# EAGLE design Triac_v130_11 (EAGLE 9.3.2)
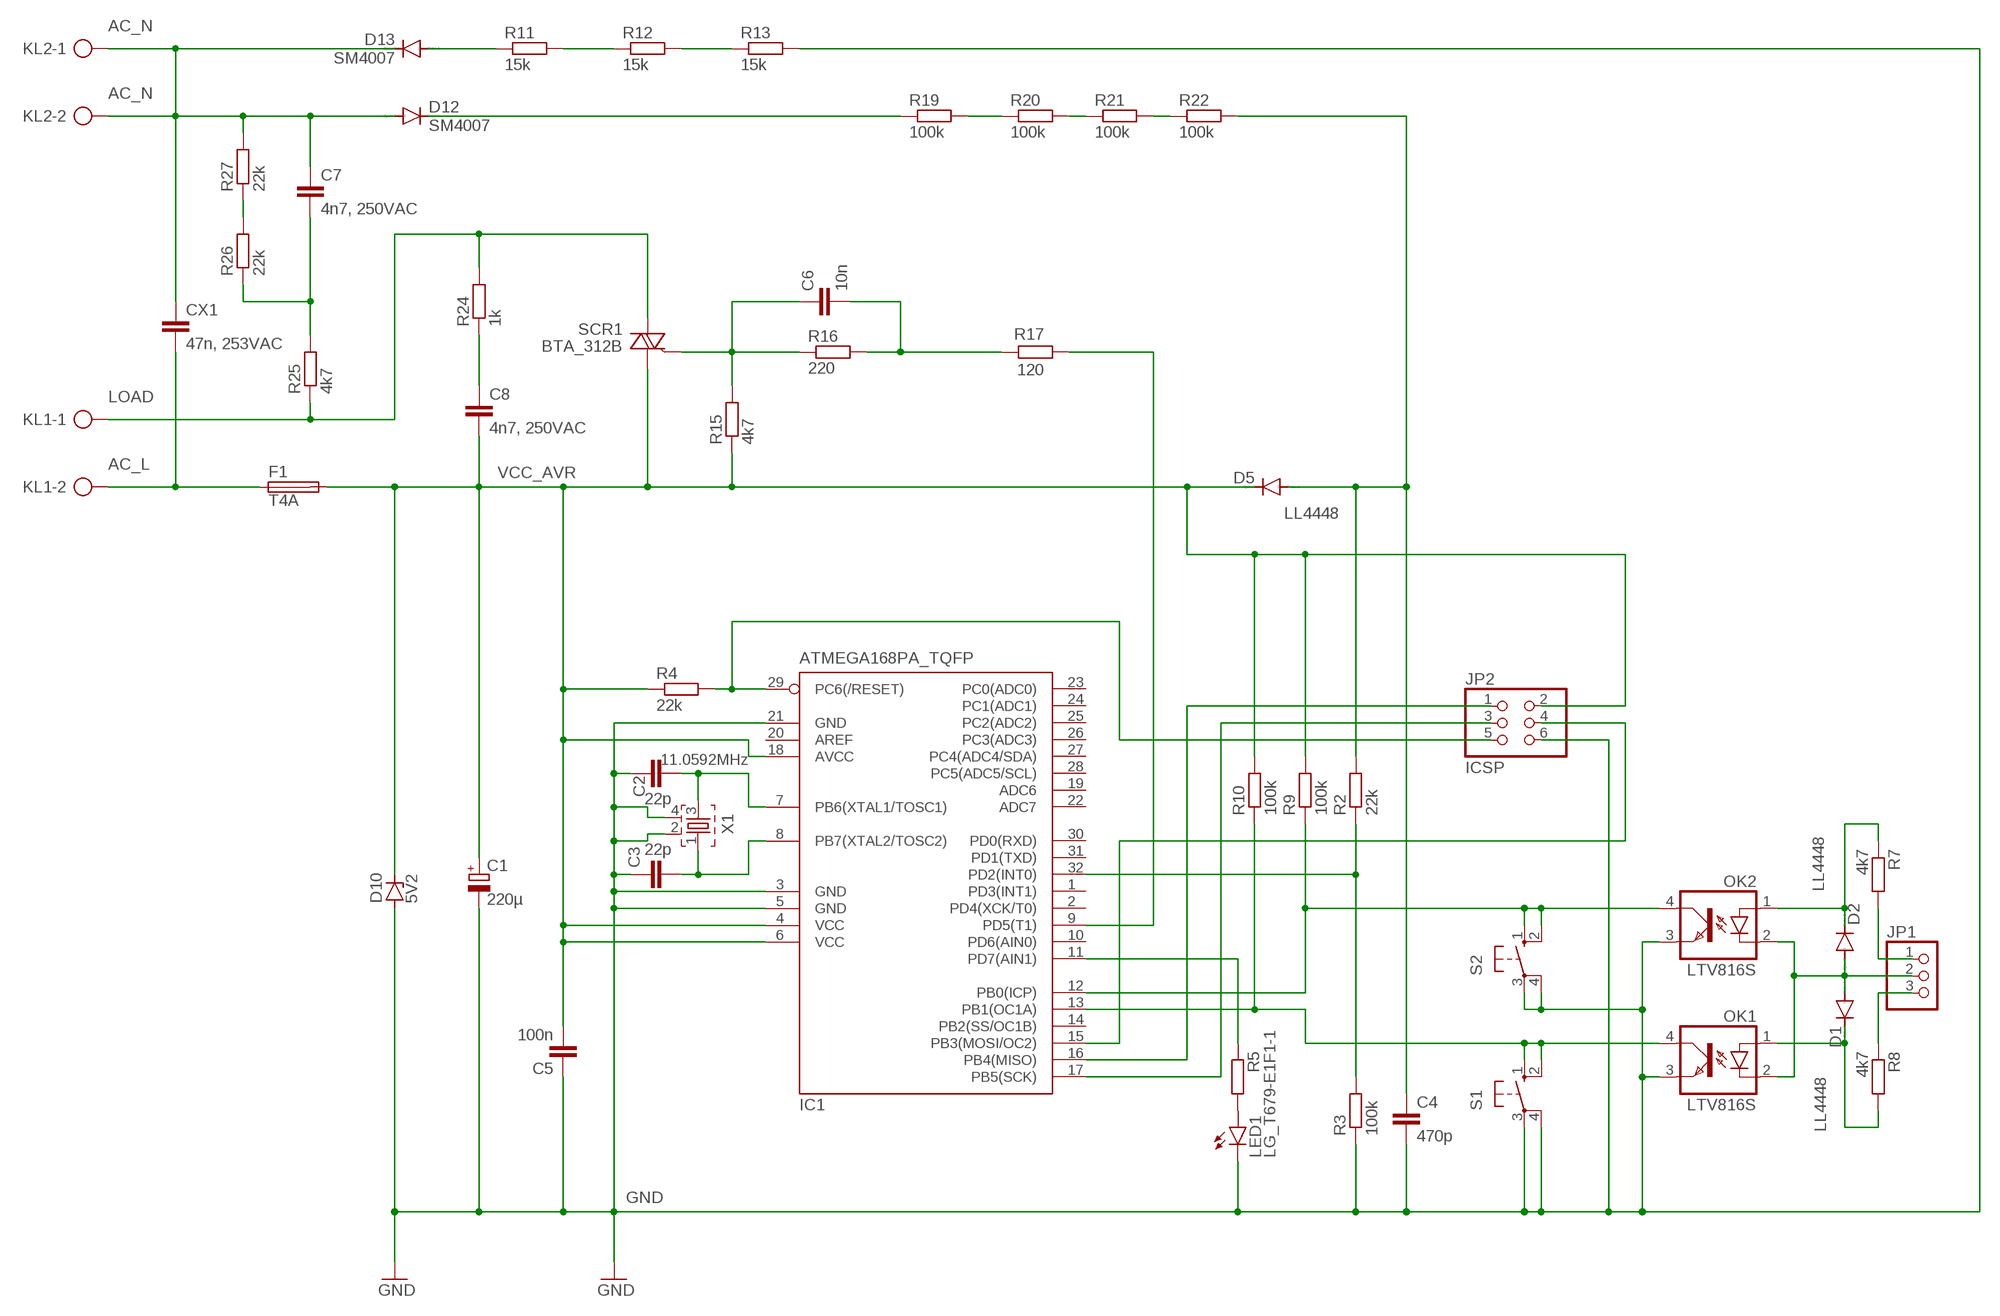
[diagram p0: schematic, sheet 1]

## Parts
C1  220µ  CPOL-EU153CLV-0605  [153CLV-0605]
C2  22p  C-EUC0805  [C0805]
C3  22p  C-EUC0805  [C0805]
C4  470p  C-EUC0805  [C0805]
C5  100n  C-EUC0805  [C0805]
C6  10n  C-EUC0805K  [C0805K]
C7  4n7, 250VAC  C5/3  [C5B3]
C8  4n7, 250VAC  C5/3  [C5B3]
CX1  47n, 253VAC  XC_03  [XC22B6]
D1  LL4448  [SOD80C]
D2  LL4448  [SOD80C]
D5  LL4448  [SOD80C]
D10  5V2  ZENER-DIODESOD80C  [SOD80C]
D12  SM4007  DIODE-DO214AA  [DO214AA]
D13  SM4007  DIODE-DO214AA  [DO214AA]
F1  T4A  SHK20QPADS  [SHK20Q]
IC1  ATMEGA168PA_TQFP  MEGA8-AI  [TQFP32-08]
JP1  PINHD-1X3  [1X03]
JP2  ICSP  PIN2X3  [2X03]
KL1  2pole-7.5mm  KL2_75  [KL2-75]
KL2  KL2_75  [KL2-75]
LED1  LG_T679-E1F1-1  [PLCC2]
OK1  LTV816S  [DIL4-SMD]
OK2  LTV816S  [DIL4-SMD]
R2  22k  R-EU_R0805  [R0805]
R3  100k  R-EU_R0805  [R0805]
R4  22k  R-EU_R0805  [R0805]
R5  R-EU_R0805  [R0805]
R7  4k7  R-EU_R0805  [R0805]
R8  4k7  R-EU_R0805  [R0805]
R9  100k  R-EU_R0805  [R0805]
R10  100k  R-EU_R0805  [R0805]
R11  15k  R-EU_MELF0207R  [MINI_MELF-0207R]
R12  15k  R-EU_MELF0207R  [MINI_MELF-0207R]
R13  15k  R-EU_MELF0207R  [MINI_MELF-0207R]
R15  4k7  R-EU_R0805  [R0805]
R16  220  R-EU_R0805  [R0805]
R17  120  R-EU_R0805  [R0805]
R19  100k  R-EU_R0805  [R0805]
R20  100k  R-EU_R0805  [R0805]
R21  100k  R-EU_R0805  [R0805]
R22  100k  R-EU_R0805  [R0805]
R24  1k  R-EU_MELF0207R  [MINI_MELF-0207R]
R25  4k7  R-EU_MELF0207R  [MINI_MELF-0207R]
R26  22k  R-EU_MELF0207R  [MINI_MELF-0207R]
R27  22k  R-EU_MELF0207R  [MINI_MELF-0207R]
S1  10-XX  [B3F-10XX]
S2  10-XX  [B3F-10XX]
SCR1  BTA_312B  [D2PACK]
X1  11.0592MHz  406_NEW  [CTS406]

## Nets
AC_L: CX1.2 F1.1A F1.1B KL1.2
AC_N: C7.1 CX1.1 D12.A D13.C KL2.1 KL2.2 R27.2
GND: C1.- C2.1 C3.1 C4.2 C5.1 D10.A IC1.3(GND) IC1.5(GND) IC1.21(GND) JP2.6 LED1.C OK1.3(EMIT) OK2.3(EMIT) R3.1 R13.2 S1.3(P) S1.4(P1) S2.3(P) S2.4(P1) X1.2 X1.4
LOAD: KL1.1 R24.2 R25.1 SCR1.T2(A2)
N$1: C2.2 IC1.7(PB6(XTAL1/TOSC1)) X1.3
N$3: IC1.11(PD7(AIN1)) R5.1
N$4: R26.2 R27.1
N$5: D13.A R11.1
N$6: R11.2 R12.1
N$7: R12.2 R13.1
N$8: C6.1 R15.2 R16.1 SCR1.G
N$9: D12.C R19.1
N$10: R19.2 R20.1
N$11: R20.2 R21.1
N$12: R21.2 R22.1
N$13: C6.2 R16.2 R17.2
N$14: C3.2 IC1.8(PB7(XTAL2/TOSC2)) X1.1
N$15: C7.2 R25.2 R26.1
N$16: C4.1 D5.A R2.2 R22.2
N$17: IC1.29(PC6(/RESET)) JP2.5 R4.2
N$18: C8.1 R24.1
N$19: IC1.12(PB0(ICP)) OK2.4(COL) R9.1 S2.1(S) S2.2(S1)
N$23: IC1.17(PB5(SCK)) JP2.3
N$24: LED1.A R5.2
N$25: IC1.9(PD5(T1)) R17.1
N$26: IC1.13(PB1(OC1A)) OK1.4(COL) R10.1 S1.1(S) S1.2(S1)
N$27: JP1.1 R7.2
N$28: IC1.32(PD2(INT0)) R2.1 R3.2
N$29: D2.C OK2.1(A) R7.1
N$30: JP1.3 R8.1
N$31: D1.C OK1.1(A) R8.2
N$32: IC1.16(PB4(MISO)) JP2.1
N$34: D1.A D2.A JP1.2 OK1.2(C) OK2.2(C)
N$36: IC1.15(PB3(MOSI/OC2)) JP2.4
VCC_AVR: C1.+ C5.2 C8.2 D5.C D10.C F1.2A F1.2B IC1.4(VCC) IC1.6(VCC) IC1.18(AVCC) JP2.2 R4.1 R9.2 R10.2 R15.1 SCR1.T1(A1)
Unconnected: IC1.1(PD3(INT1)) IC1.2(PD4(XCK/T0)) IC1.10(PD6(AIN0)) IC1.14(PB2(SS/OC1B)) IC1.19(ADC6) IC1.20(AREF) IC1.22(ADC7) IC1.23(PC0(ADC0)) IC1.24(PC1(ADC1)) IC1.25(PC2(ADC2)) IC1.26(PC3(ADC3)) IC1.27(PC4(ADC4/SDA)) IC1.28(PC5(ADC5/SCL)) IC1.30(PD0(RXD)) IC1.31(PD1(TXD))

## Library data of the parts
C1 = rcl:CPOL-EU: POLARIZED CAPACITOR, European symbol; SPICEPREFIX: C
C2-C6 = rcl:C-EU: CAPACITOR, European symbol; SPICEPREFIX: C
C7 C8 = capacitor-wima:C: CAPACITOR
CX1 = MY_CX:XC_03: Device XC_03
D1 D2 D5 = My_Diode:LL4448
D10 = diode:ZENER-DIODE: Z-Diode
D12 D13 = diode:DIODE-: DIODE
F1 = MY_Fuse:SHK20Q: FUSE HOLDER
IC1 = atmel:MEGA8: MICROCONTROLLER 8 Kbytes FLASH, 1 kbytes SRAM, 512 bytes EEPROM, USART, 6-channel 10 bit ADC, 2-channel 8 bit ADC Pin compatible with Atmega48, ATMega88, ATMega168 Source: avr.lbr; MPN: ATMEGA8-16AU; OC_FARNELL: 9171371; OC_NEWARK: 73M8863
JP1 = pinhead:PINHD-1X3: PIN HEADER
JP2 = pinhead_2x3:PIN2X3
KL1 KL2 = MY_Clamp_1:KL2_75: 2-pole Screw Terminal
LED1 = led:*_T679-?-1: LC TOPLED® Low Current LED; COLOR: green
OK1 OK2 = optocoupler:LTV816: OPTO COUPLER Source: LITEON, LTV816.pdf
R2-R5 R7-R13 R15-R17 R19-R22 R24-R27 = rcl:R-EU_: RESISTOR, European symbol; SPICEPREFIX: R
S1 S2 = switch-omron:10-XX: OMRON SWITCH; MPN: B3F-1000; OC_FARNELL: 176432; OC_NEWARK: 36M3542
SCR1 = BTA312B:BTA_312B
X1 = My_Crystal1:406_NEW

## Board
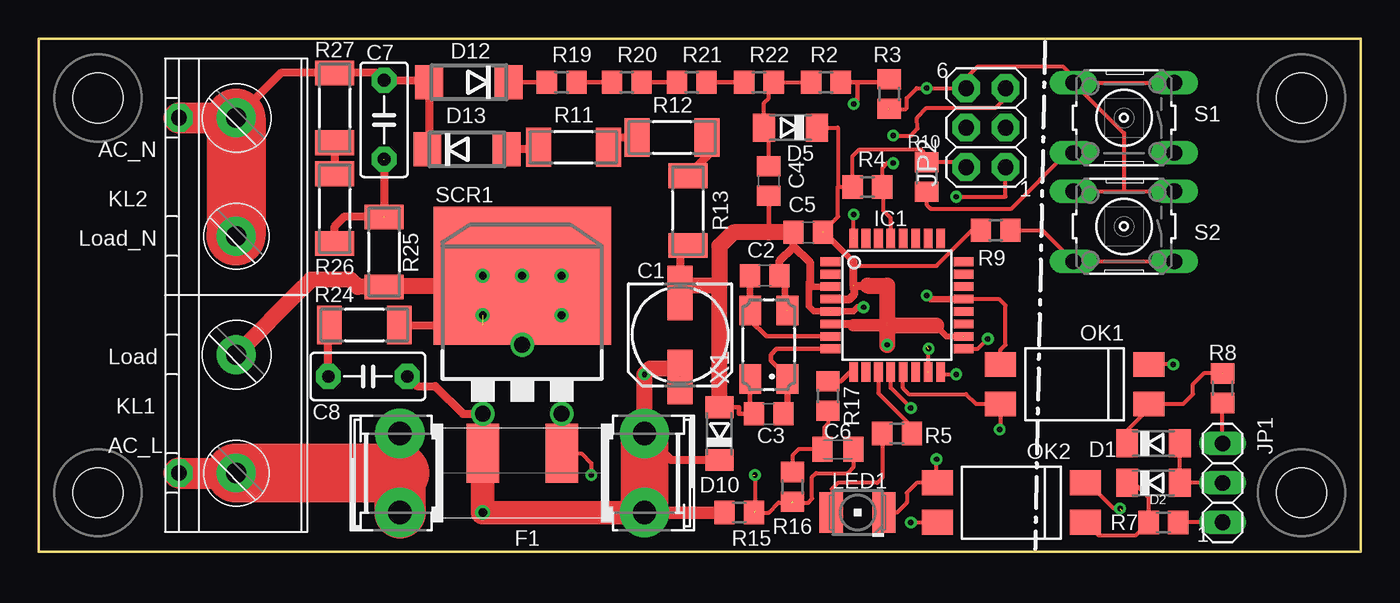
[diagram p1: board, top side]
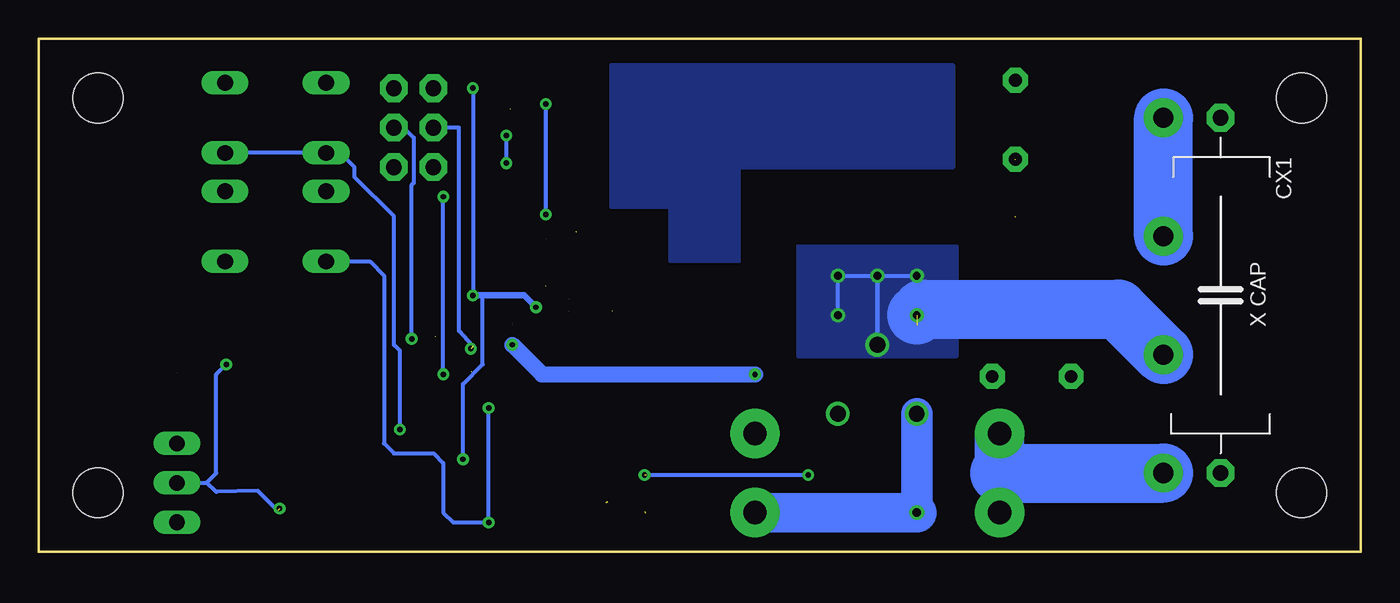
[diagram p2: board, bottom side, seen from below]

Size 85.09 x 33.02 mm. Coordinates in mm from the lower left corner, seen from the top.
Outline: 0,33.02 0,0 85.09,0 85.09,33.02 0,33.02
Copper layers (1*16): Top 0.035mm / dielectric 1.5mm / Bottom 0.035mm
Design rules "default *": minimum track width 10mil, minimum drill 0.35mm, track to track 6mil, track to pad 6mil, pad to pad 6mil, via to via 6mil, smd to smd 6mil, copper to edge 30mil, drill to drill 6mil, minimum pad ring 10mil, minimum via ring 8mil, stop-mask expansion 6mil, vias tented up to drill 0mil, thermal gap 10mil
Holes 3.2 mm at 81.28,3.81 81.28,29.21 3.81,3.81 3.81,29.21

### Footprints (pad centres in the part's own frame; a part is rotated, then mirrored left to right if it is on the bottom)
153CLV-0605 = smd 3.5 x 1.6: + 2.7,0; - -2.7,0
C0805 = smd 1.3 x 1.5: 1 -0.95,0; 2 0.95,0
C0805K = smd 1.3 x 1.6: 1 -1,0; 2 1,0
C5B3 = drill 0.813 pad 1.6 octagon: 1 -2.54,0; 2 2.54,0
XC22B6 = drill 1.016 pad 1.778 octagon: 1 -11.43,0; 2 11.43,0
SOD80C = smd 1.4 x 1.8: A 1.7,0; C -1.7,0
DO214AA = smd 1.8 x 2.2: A 2.55,0; C -2.55,0
SHK20Q = drill 1.5 pad 3.175: 1A -7.874,2.54; 1B -7.874,-2.54; 2A 7.874,2.54; 2B 7.874,-2.54
TQFP32-08 = smd 1.27 x 0.559: 1 -4.293,2.8; 2 -4.293,2; 3 -4.293,1.2; 4 -4.293,0.4; 5 -4.293,-0.4; 6 -4.293,-1.2; 7 -4.293,-2; 8 -4.293,-2.8; 17 4.293,-2.8; 18 4.293,-2; 19 4.293,-1.2; 20 4.293,-0.4; 21 4.293,0.4; 22 4.293,1.2; 23 4.293,2; 24 4.293,2.8 | smd 0.559 x 1.27: 9 -2.8,-4.293; 10 -2,-4.293; 11 -1.2,-4.293; 12 -0.4,-4.293; 13 0.4,-4.293; 14 1.2,-4.293; 15 2,-4.293; 16 2.8,-4.293; 25 2.8,4.293; 26 2,4.293; 27 1.2,4.293; 28 0.4,4.293; 29 -0.4,4.293; 30 -1.2,4.293; 31 -2,4.293; 32 -2.8,4.293
1X03 = drill 1.016 long: 1 -2.54,0; 2 0,0; 3 2.54,0
2X03 = drill 1.016 pad 1.778 octagon: 1 -2.54,-1.27; 2 -2.54,1.27; 3 0,-1.27; 4 0,1.27; 5 2.54,-1.27; 6 2.54,1.27
KL2-75 = drill 1.3 pad 2.5: 1 -3.81,0; 2 3.81,0
PLCC2 = smd 2.6 x 1.5: A 0,1.7; C 0,-1.7
DIL4-SMD = smd 1.6 x 2: 1 -1.27,-4.77; 2 1.27,-4.77; 3 1.27,4.77; 4 -1.27,4.77
R0805 = smd 1.3 x 1.5: 1 -0.95,0; 2 0.95,0
MINI_MELF-0207R = smd 1.6 x 2.5: 1 -2.25,0; 2 2.25,0
B3F-10XX = drill 1.016 long: 1 -3.251,2.261; 2 3.251,2.261; 3 -3.251,-2.261; 4 3.251,-2.261
D2PACK = smd 2.083 x 3.81: G 2.54,-7.62; T1 -2.54,-7.62 | smd 11.43 x 8.89: T2 0,3.81
CTS406 = smd 1.9 x 1.4: 1 -2.2,-1.2; 2 2.2,-1.2; 3 2.2,1.2; 4 -2.2,1.2

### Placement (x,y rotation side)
C1  41.27,13.97 270 top
C2  46.74,17.78 180 top
C3  46.99,8.89 0 top
C4  46.99,23.88 270 top
C5  49.53,20.57 0 top
C6  51.44,6.6 180 top
C7  22.23,27.81 270 top
C8  21.18,11.3 0 top
CX1  9.02,16.51 270 bottom
D1  71.75,6.99 0 top
D2  71.75,4.45 0 top
D5  48.39,27.3 180 top
D10  43.81,7.62 90 top
D12  27.69,30.23 180 top
D13  27.56,25.91 0 top
F1  31.11,5.08 0 top
IC1  55.24,15.88 0 top
JP1  76.2,4.45 90 top
JP2  60.96,27.3 90 top
KL1  12.7,8.89 270 top
KL2  12.7,24.13 270 top
LED1  52.7,2.54 90 top
OK1  66.67,10.79 90 top
OK2  62.61,3.17 90 top
R2  50.67,30.23 180 top
R3  54.74,29.46 90 top
R4  53.34,23.5 0 top
R5  55.24,7.62 180 top
R7  72.39,1.91 0 top
R8  76.2,10.54 90 top
R9  61.59,20.7 180 top
R10  57.15,24.13 90 top
R11  34.42,26.04 0 top
R12  40.77,26.67 0 top
R13  41.78,21.97 270 top
R15  45.09,2.54 0 top
R16  48.51,4.19 90 top
R17  50.8,10.03 270 top
R19  33.66,30.23 0 top
R20  37.85,30.23 0 top
R21  42.04,30.23 0 top
R22  46.35,30.23 0 top
R24  20.95,14.61 0 top
R25  22.23,19.3 90 top
R26  19.05,22.1 90 top
R27  19.05,28.57 90 top
S1  69.85,27.94 180 top
S2  69.85,20.95 180 top
SCR1  31.11,13.97 0 top
X1  46.99,13.34 90 top

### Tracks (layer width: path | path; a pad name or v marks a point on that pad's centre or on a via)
AC_L
  Top 2: CX1.2 KL1.2
  Top 3.302: F1.1B 23.24,5.08
  Top 3.81: 23.24,5.08 KL1.2
  Bottom 3.175: F1.1A 23.24,5.08
  Bottom 3.81: 23.24,5.08 KL1.2
AC_N
  Top 0.508: 13.02,28.26 15.59,30.82 R27.2 21.74,30.82 22.21,30.35 C7.1 25.01,30.35 D12.A 25.14,26.04
  Top 0.61: 25.14,26.04 D13.C
  Top 2: CX1.1 KL2.1
  Top 2.54: KL2.1 13.02,28.26
  Top 3.81: KL2.1 KL2.2
  Bottom 3.81: KL2.2 KL2.1
GND  (via drill 0.35)  (3 unrouted)
  Top 0.254: 54.74,28.48 55.75,28.48 55.87,28.58 55.88,29.21 56.52,29.84 v57.15,29.84 JP2.6 59.69,30.48 60.45,31.24 65.91,31.24 66.67,30.48 66.67,30.28 S1.4 | OK1.3 61.91,13.01 62.23,13.34 62.23,15.88 61.85,16.26 59.56,16.26 IC1.21 | v57.78,5.97 57.78,4.5 OK2.3 56.52,4.45 55.88,3.81 55.88,3.17 55.24,2.54 LED1.C | S2.4 69.85,23.22 | 69.85,23.22 S2.3 | S1.4 S1.3 | S1.4 69.85,26.95 69.85,23.22 | IC1.5 50.95,15.49 51.44,15.49 | C2.1 48.03,17.78 | R13.2 41.78,19.21 41.27,19.21
  Top 0.305: C4.2 46.99,20.57 | D10.A 45.09,9.32 45.09,8.89 45.72,8.89 45.79,8.89 | 45.79,8.89 C3.1 | X1.4 45.79,8.89
  Top 0.406: v57.15,16.51 57.38,16.27 IC1.21 | v53.09,15.75 52.7,15.75 52.45,15.49 51.44,15.49 | IC1.3 49.85,17.07 49.66,17.27 49.58,17.35 49.58,15.82 49.91,15.49 50.95,15.49 | 48.16,15.54 48.03,16.64 48.03,17.78
  Top 0.508: C2.1 47.69,18.73 48.58,19.62 48.58,19.68 | 48.58,19.68 C5.1 | 41.27,19.21 C1.- | 49.66,17.27 49.66,18.61 48.58,19.68
  Top 0.61: 41.75,17.14 C1.-
  Top 1.016: C5.1 46.99,20.57 44.7,20.57 43.81,19.68 43.81,17.14 | 43.81,17.14 41.75,17.14 | D10.A 43.81,17.14
  Bottom 0.254: v57.15,29.84 v57.15,16.51 | v57.78,5.97 57.78,10.79 56.52,12.06 56.52,16.51
  Bottom 0.406: v57.15,16.51 56.52,16.51 53.85,16.51 v53.09,15.75
LOAD  (via drill 0.5, 1.02)  (1 unrouted)
  Top 0.305: 30.48,17.78 SCR1.T2
  Top 0.508: R24.2 28.57,14.61
  Top 1.016: KL1.1 17.05,17.05 17.14,17.14 17.27,17.27 17.53,17.53 20.07,17.53 20.54,17.05 R25.1 22.32,17.14 27.94,17.14
  Bottom 0.254: v33.66,15.24 v33.66,17.78 SCR1.T2 v28.57,17.78 v28.57,15.24
  Bottom 0.305: SCR1.T2 v31.11,13.34
  Bottom 3.81: v28.57,15.24 28.19,15.62 15.62,15.62 KL1.1
  other vias: 31.11,17.78
  pour Bottom (isolate 1.016): 36.2,19.68 26.04,19.68 26.04,12.57 36.2,12.57
N$1
  Top 0.305: IC1.7 46.83,13.88 45.79,14.92 X1.3
  Top 0.406: X1.3 C2.2
  Top 0.508: C2.2
N$2
  pour Bottom: 26.23,24.77 26.23,31.31 48.26,31.31 48.26,22.23 44.45,22.23 44.45,18.73 40.01,18.73 40.01,24.77
N$3
  Top 0.254: IC1.11 54.05,10.22 56.2,8.07 R5.1
N$4
  Top 0.508: R27.1 R26.2
N$5
  Top 0.508: R11.1 32.04,25.91 D13.A
N$6
  Top 0.508: R12.1 37.3,26.67 R11.2
N$7
  Top 0.508: R12.2 43.02,25.45 R13.1
N$8  (via drill 0.35, 1.02)  (4 unrouted)
  Top 0.254: SCR1.G 34.92,6.35 35.56,5.71 v35.56,4.95 | v46.1,4.95 46.1,2.61 | R15.2 46.99,2.54 47.62,3.17 48.45,3.17 | C6.1 52.44,5.45 52.07,5.08 50.04,5.08 49.78,4.83 49.78,3.43 49.53,3.17 48.58,3.17
  Top 0.508: v33.66,8.89 SCR1.G
  Bottom 0.254: v35.56,4.95 45.97,4.95
N$9
  Top 0.305: D12.C R19.1
N$10
  Top 0.305: R19.2 R20.1
N$11
  Top 0.305: R20.2 R21.1
N$12
  Top 0.305: R21.2 R22.1
N$13
  Top 0.254: R17.2 50.8,8.26 50.55,8 50.55,6.99 | 50.16,6.6 48.9,6.6 48.51,6.22 R16.2
  Top 0.305: 50.16,6.6 C6.2 50.44,6.99 50.55,6.99
N$14
  Top 0.254: 48.19,9.14 C3.2
  Top 0.305: IC1.8 47.5,13.07 47.5,13.08 47.12,12.7 47.12,12.32 48.19,11.25 X1.1
  Top 0.406: X1.1 48.19,9.14
N$15  (2 unrouted)
  Top 0.508: R26.1 19.05,20.95 19.68,21.59 22.23,21.59 22.23,25.26
N$16
  Top 0.254: R2.2 R22.2 46.99,30.23 46.99,29.21 46.69,28.91 46.69,27.94 D5.A | C4.1 46.99,27 D5.A | D5.A
N$17  (via drill 0.35)
  Top 0.254: v54.99,26.8 56.13,26.8 56.56,27.26 56.53,27.94 57.15,28.57 61.59,28.57 62.23,29.21 JP2.5 | IC1.29 54.84,21.48 54.36,21.97 54.36,23.43 R4.2 54.29,24.7 54.61,25.02 v54.99,25.02
  Bottom 0.254: v54.99,25.02 v54.99,26.8
N$18
  Top 0.254: 18.64,14.54 R24.1
  Top 0.508: C8.1 18.64,14.54
N$19  (via drill 0.35)
  Top 0.254: S2.1 S2.2 64.59,20.7 R9.1 | v56.13,1.91 OK2.4 | v56.13,9.27 54.84,10.56 IC1.12
  Bottom 0.254: S2.2 63.78,18.69 62.87,17.78 62.87,6.99 62.23,6.35 59.69,6.35 59.05,5.71 59.05,2.54 58.42,1.91 v56.13,1.91 v56.13,9.27
N$23  (via drill 0.35)
  Top 0.254: IC1.17 60.45,13.08 v61.09,13.72
  Bottom 0.254: v61.09,13.72 61.09,23.62 60.96,23.75 60.96,26.67 61.59,27.3 JP2.3
N$24
  Top 0.254: R5.2 54.3,4.76 53.98,4.45 51.44,4.45 51.05,4.06 51.05,2.59 LED1.A
N$25
  Top 0.254: IC1.9
  Top 0.305: R17.1 51.62,10.98 52.22,11.58 IC1.9
N$26  (via drill 0.35)
  Top 0.254: IC1.13 55.63,11.56 55.63,10.54 56.01,10.16 59.69,10.16 60.33,9.53 OK1.4 61.91,7.95 61.98,7.87 v61.85,7.87 | R10.1 57.15,22.35 57.4,22.1 62.61,22.1 66.19,25.68 S1.2
  Bottom 0.254: v61.85,7.87 61.85,12.95 62.23,13.34 62.23,21.59 64.77,24.13 64.77,24.77 65.68,25.68 S1.2 S1.1
N$27
  Top 0.254: JP1.1 R7.2
N$28  (via drill 0.35)  (2 unrouted)
  Top 0.254: IC1.32 v52.45,21.72
  Top 0.305: R2.1 52.7,30.23 | 52.7,30.23 54.55,30.23 R3.2 | v52.45,28.83 52.7,29.08 52.7,30.23
  Bottom 0.254: v52.45,21.72 v52.45,28.83
N$29
  Top 0.254: OK2.1 68.19,1.09 70.63,1.09 R7.1 71.44,3.49 70.48,4.45 D2.C
N$30
  Top 0.254: JP1.3 R8.1
N$31  (1 unrouted)
  Top 0.254: D1.C 70.06,7.83 71.44,9.21 OK1.1 73.66,9.53 74.3,10.16 74.3,10.79 74.99,11.49 75.56,11.49 | R8.2 75.56,11.49 | 75.56,11.49
N$32  (via drill 0.35)
  Top 0.254: IC1.16 58.2,11.43 v59.05,11.43 | v59.05,22.86 62.23,22.86 JP2.1
  Bottom 0.254: v59.05,11.43 v59.05,22.86
N$34  (via drill 0.35)  (1 unrouted)
  Top 0.254: JP1.2 D2.A D1.A | v73.03,12.06 OK1.2 | OK2.2 67.38,4.37 67.64,4.37 69.22,2.79 v69.6,2.79
  Bottom 0.254: 74.3,4.45 73.66,5.08 73.66,11.43 v73.03,12.06 | JP1.2 74.3,4.45 | 69.72,2.67 70.99,3.94 73.66,3.87 74.3,4.45
N$36  (via drill 0.35)  (3 unrouted)
  Top 0.254: 57.26,11.58 57.26,13.08
  Bottom 0.254: 57.13,13.22 58.04,14.22 58.04,27.3 JP2.4
  other vias: 57.28,13.08
VCC_AVR  (via drill 0.35, 0.55, 1.02)  (9 unrouted)
  Top 0.254: 51.44,23.5 51.44,27.3 D5.C | 50.47,20.59 51.44,21.57 51.44,23.5 | 52.45,18.41 57.78,18.41 60.07,20.7 R9.2 | JP2.2 59.38,25.08 R10.2 57.15,25.53 56.77,25.91 52.83,25.91 52.39,25.47 R4.1 52.07,23.5 51.44,23.5
  Top 0.406: 52.45,18.67 50.51,20.6 | 59.54,13.86 58.43,13.87 57.75,14.59 | 54.61,14.61 54.55,14.67
  Top 0.508: IC1.4 52.2,16.27 52.5,16.59 52.47,17.14 | 52.45,18.67 52.45,18.41 52.45,17.14 53.34,17.14 | F1.2A 40.69,5.92 D10.C | IC1.6 52.38,14.68 52.45,14.61 | SCR1.T1 v28.57,8.89 27.3,8.89 25.52,10.68 24.34,10.68 C8.2
  Top 0.813: F1.2B R15.1 | 52.45,14.61 54.61,14.61
  Top 1.016: F1.2A v38.99,11.43 39.37,11.81 40.73,11.81 C1.+ | 53.34,17.14 54.61,17.14 54.61,14.73 | 54.61,14.73 54.55,14.67 | 54.61,14.59 57.75,14.59 | 54.61,14.73 v54.61,13.34
  Top 1.524: SCR1.T1 v28.57,2.54 F1.2B
  Top 3.048: F1.2A F1.2B
  Bottom 1.016: v54.61,13.34 52.7,11.43 v38.99,11.43
  Bottom 2.032: v28.57,2.54 v28.57,8.89
  Bottom 2.54: F1.2B v28.57,2.54

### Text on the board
tPlace: 6 | 1 | 1
tNames: AC_N | Load_N | Load | AC_L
